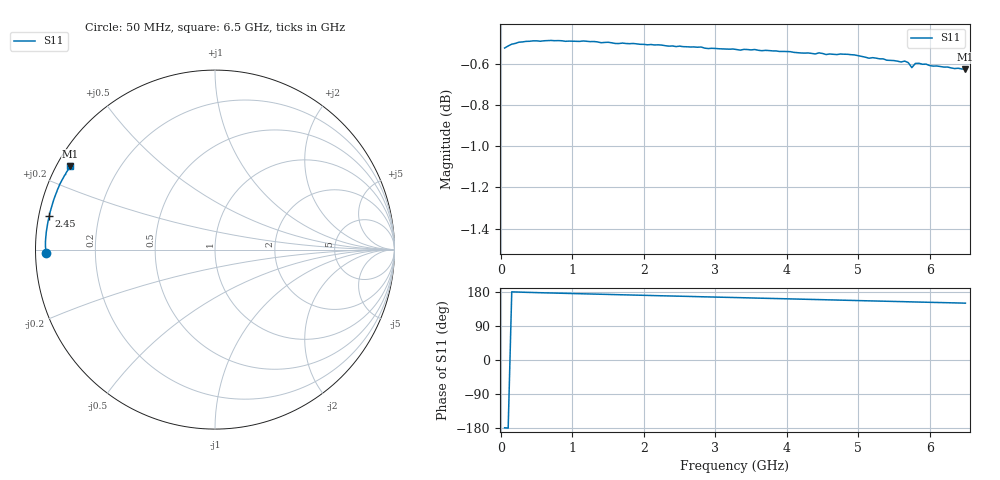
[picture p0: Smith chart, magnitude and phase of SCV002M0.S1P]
! Infineon Technologies  Discrete & RF Semiconductors
! BAR63-02L
! Si PIN Diode in TSLP-2
! IF = 2 mA
! S-Parameters:  March  2002
# GHz  S  MA  R  50
!  f  S11
! GHz  MAG  ANG
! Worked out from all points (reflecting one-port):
!   130 points, 50 MHz to 6.5 GHz, reference 50 ohm
!   lowest |S11| = -0.6 dB at 6.5 GHz (marker M1), VSWR 27.80, Z = 1.93 + j13.4 ohm
!   phase of S11 starts at -179 deg and turns -31 deg over the sweep
!   S11 on the Smith chart (normalised r, x): 50 MHz: 0.03, -0.01; 2.45 GHz: 0.03, +0.10; 6.5 GHz: 0.04, +0.27
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0.05  0.9416 -178.9
0.1  0.9427 -179.7
0.2  0.9441 179.5
0.35  0.9452 178.6
0.5  0.9454 177.9
0.6  0.9455 177.3
0.7  0.9456 176.9
0.9  0.9452 175.9
1.2  0.9452 174.4
1.7  0.9443 172.1
2.15  0.9433 170.0
2.2  0.9433 169.7
2.45  0.9424 168.6
2.5  0.9426 168.3
2.65  0.9422 167.7
2.85  0.9416 166.7
3  0.9414 166.1
3.05  0.9413 165.8
3.3  0.9408 164.7
4  0.9398 161.4
4.1  0.9394 161.0
4.9  0.9381 157.3
5.05  0.9372 156.5
5.7  0.934 153.6
5.75  0.9314 153.3
5.8  0.9336 153.1
5.95  0.9332 152.5
6.5  0.9305 150.0
